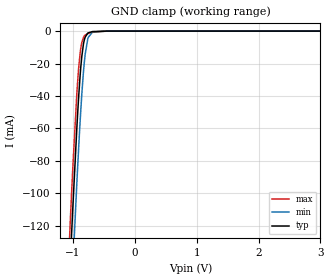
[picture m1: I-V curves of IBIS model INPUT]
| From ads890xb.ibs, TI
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|   INPUT
[Model]   INPUT
Model_type   Input
Vinl = 0.56
Vinh = 2.24
|   typ   min   max
C_comp   3.81628E-13  3.71228E-13  3.85159E-13
[Model spec]
|subparameter
Vinl   0.36   0.33   0.47
Vinh   1.44   1.32   1.88
|Where Nom  PVT is Nominal Process,  1.8V, 25C
|   Fast PVT is Strong Process,  2.35V, 0C
|   Slow PVT is Weak Process,   1.65V, 60C
[Voltage Range]   1.8   1.65   2.35
[Temperature Range]   25   60   0
[Power Clamp Reference]   1.8   1.65   2.35
[GND Clamp Reference]   0   0   0
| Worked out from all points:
|   GND clamp passes 1 mA (typ) near -0.74 V on its own axis
[GND Clamp]
|   Voltage   I(typ)   I(min)   I(max)
-1.8V     -855.5mA   -893.5mA   -829.3mA
-1.174V   -259.8mA   -298.7mA   -233mA
-1.039V   -140.7mA   -178.5mA   -115mA
-1.022V   -127.2mA   -164.6mA   -101.8mA
-1.001V   -109.5mA   -146.4mA   -84.65mA
-936mV    -60.31mA   -94.33mA   -39.07mA
-882mV    -27.35mA   -55.63mA   -13.51mA
-855mV    -15.63mA   -38.98mA   -7.014mA
-817.2mV  -5.896mA   -20.29mA   -3.17mA
-752.4mV  -1.102mA   -4.015mA   -1.476mA
-444.6mV  -1.196uA   -498.8nA   -9.557uA
3.6V      0A         0A         0A
[POWER Clamp]
|   Voltage   I(typ)   I(min)   I(max)
-1.8V     0A         0A         0A
0V        0A         0A         0A
3.6V      0A         0A         0A
